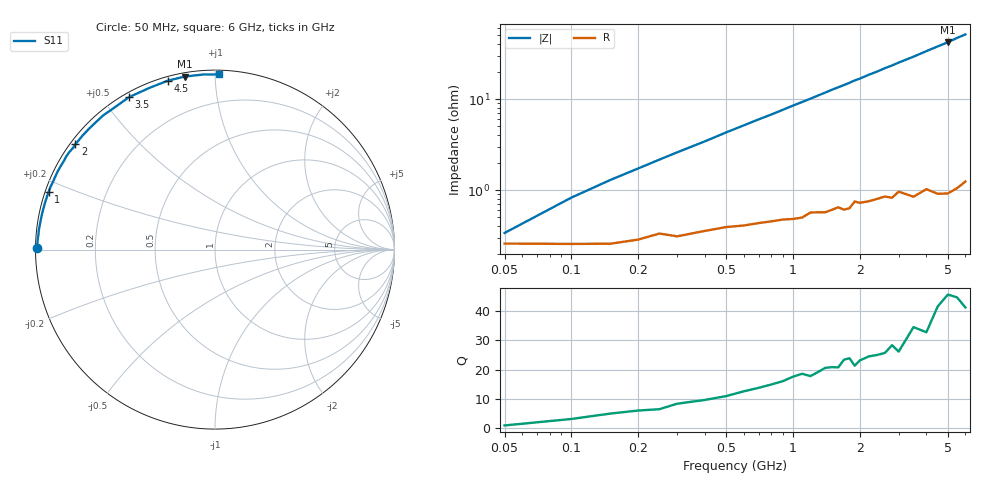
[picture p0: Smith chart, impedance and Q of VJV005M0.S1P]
! Infineon Technologies  Discrete & RF Semiconductors
! BB 914
! Si Tuning Diode in SOT23
! VR =
! S-Parameters:  July  1999
# GHz  S  MA  R  50
!  f  S11
! GHz  MAG  ANG
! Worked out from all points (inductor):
!   34 points, 50 MHz to 6 GHz, reference 50 ohm
!   read as one part to ground: L = 1.34 nH near 100 MHz
!   highest Q = 44.8 at 5 GHz (marker M1), where L = 1.34 nH
!   S11 on the Smith chart (normalised r, x): 50 MHz: 0.01, +0.00; 1 GHz: 0.01, +0.17; 2 GHz: 0.01, +0.33; 3.5 GHz: 0.02, +0.58; 4.5 GHz: 0.02, +0.76; 6 GHz: 0.02, +1.02
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0.05  0.9897 179.5
0.1  0.9898 178.2
0.15  0.9898 177.1
0.25  0.9868 175.1
0.3  0.9877 174.1
0.6  0.984 168.3
0.7  0.983 166.4
0.8  0.9823 164.6
1  0.9814 160.8
1.1  0.9809 159.0
1.4  0.9786 153.5
1.5  0.9774 151.6
1.6  0.9761 149.9
1.7  0.9777 148.2
1.8  0.9771 146.4
1.9  0.9731 144.5
2  0.9743 143.0
2.2  0.9738 139.4
2.4  0.9728 136.3
2.6  0.9719 132.8
2.8  0.9733 129.9
3  0.9698 126.6
3.5  0.9751 119.4
4  0.9722 112.2
4.5  0.9771 105.7
5  0.9787 99.9
5.5  0.978 93.6
6  0.9761 88.6
